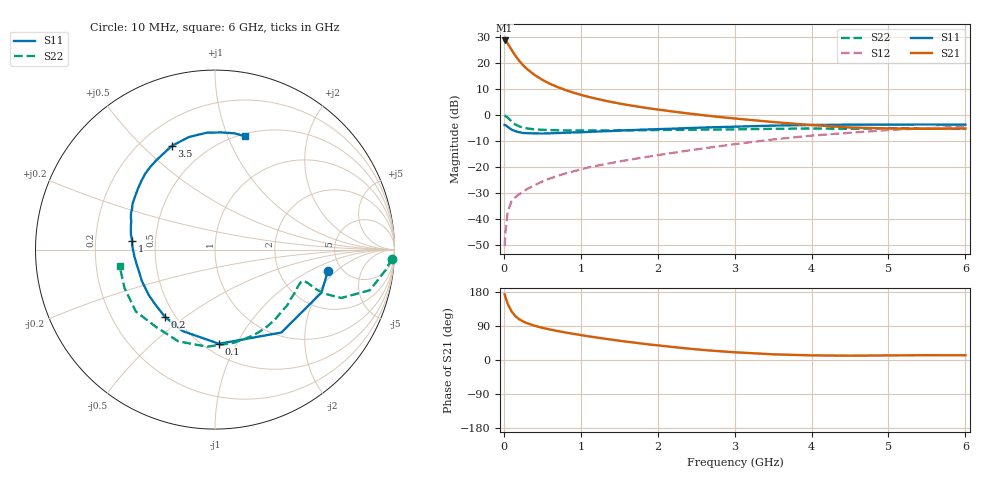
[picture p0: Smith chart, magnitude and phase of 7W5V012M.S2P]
! Infineon Technologies  Discrete & RF Semiconductors
! BFS17W
! Si NPN RF Bipolar Junction Transistor in SOT323
! VCE = 5 V  IC = 12 mA
! Common Emitter S-Parameters:  August  1999
# GHz  S  MA  R  50
!  f  S11  S21  S12  S22
! GHz  MAG  ANG  MAG  ANG  MAG  ANG  MAG  ANG
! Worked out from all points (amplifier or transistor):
!   36 points, 10 MHz to 6 GHz, reference 50 ohm
!   highest |S21| = 28.7 dB at 10 MHz (marker M1)
!   |S21| within 3 dB of that: start of sweep to 87.87 MHz
!   unconditionally stable (mu >= 1): 374.4 MHz to 2.275 GHz; 5.175 GHz to end of sweep
!   at 250 MHz: K = 0.85, MSG = 24.3 dB, |S12| = -29.5 dB
!   at 1.4 GHz: K = 1.18, MAG = 9.1 dB, |S12| = -18.5 dB
!   at 6 GHz: K = 1.05, MAG = -1.7 dB, |S12| = -4.5 dB
!   S11 on the Smith chart (normalised r, x): 10 MHz: 3.87, -1.59; 100 MHz: 0.59, -0.85; 200 MHz: 0.44, -0.42; 1 GHz: 0.37, +0.05; 3.5 GHz: 0.32, +0.62; 6 GHz: 0.53, +1.16
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0.01  0.6405 -10.9  27.19 173.4  0.003 80.7  0.9872 -2.9
0.02  0.6394 -22.1  26.87 166.3  0.0054 85.3  0.9585 -6.7
0.05  0.5919 -51.3  23.77 148.5  0.0138 72.3  0.8919 -14.7
0.1  0.5251 -87.6  17.99 128.2  0.0219 58.5  0.7526 -21.0
0.15  0.4883 -111.6  13.81 115.5  0.0262 57.1  0.657 -21.9
0.2  0.4668 -126.8  11.02 107.5  0.03 56.4  0.6053 -21.4
0.25  0.4516 -137.5  9.075 101.7  0.0336 56.4  0.5716 -20.5
0.3  0.4478 -145.5  7.699 97.3  0.0376 58.6  0.5537 -19.9
0.4  0.4434 -157.0  5.892 90.3  0.0446 60.9  0.5298 -19.4
0.5  0.4409 -164.6  4.761 85.0  0.0525 62.9  0.5203 -19.6
0.6  0.4449 -170.4  3.984 80.5  0.0601 64.7  0.5134 -20.4
0.7  0.4504 -175.1  3.446 76.4  0.0675 66.1  0.5092 -21.6
0.8  0.4565 -179.5  3.032 72.6  0.0752 66.8  0.5066 -23.2
1  0.4648 173.8  2.449 65.9  0.0897 67.9  0.5068 -26.5
1.1  0.4747 170.2  2.238 62.5  0.0982 68.4  0.5053 -28.8
1.6  0.511 156.3  1.568 48.2  0.1353 69.8  0.5063 -40.4
2.2  0.5465 142.0  1.166 34.2  0.1874 71.1  0.5179 -56.4
2.8  0.5855 127.9  0.918 23.2  0.251 69.4  0.5261 -73.7
3.5  0.6261 112.6  0.733 15.0  0.3385 64.3  0.5429 -94.7
4.5  0.6529 94.0  0.575 11.4  0.4558 52.0  0.5419 -127.4
5.5  0.6569 80.3  0.542 12.7  0.5587 39.1  0.5477 -157.0
6  0.6528 75.2  0.552 12.5  0.5989 32.7  0.5391 -170.2
